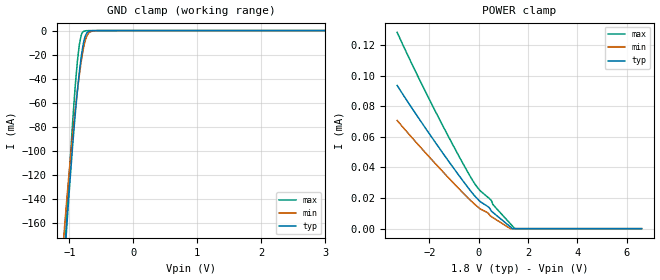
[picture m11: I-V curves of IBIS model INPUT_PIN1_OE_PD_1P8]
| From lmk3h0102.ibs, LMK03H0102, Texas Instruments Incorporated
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[Model]   INPUT_PIN1_OE_PD_1P8
Model_type   Input
Vinl = 0.65
Vinh = 1.15
|   typ   min   max
C_comp   0.7pF   0.5pF   0.9pF
[Voltage Range]   1.8   1.71   1.89
[Temperature Range]   45   125   -40
[Power Clamp Reference]   1.8   1.71   1.89
[GND Clamp Reference]   0   0   0
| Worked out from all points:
|   GND clamp passes 1 mA (typ) near -0.71 V on its own axis
[GND Clamp]
|   Voltage   I(typ)   I(min)   I(max)
-3.3V     -2.163A    -1.946A    -2.393A
-1.142V   -244.3mA   -209.2mA   -247.1mA
-1.073V   -188.3mA   -161.6mA   -183.1mA
-1.043V   -165mA     -142.2mA   -156.3mA
-943.8mV  -92.69mA   -84.35mA   -72.63mA
-874.5mV  -50.33mA   -50.21mA   -25.69mA
-844.8mV  -35.17mA   -37.37mA   -12.01mA
-815.1mV  -22.23mA   -25.95mA   -4.039mA
-765.6mV  -7.235mA   -11.31mA   -401.3uA
-696.3mV  -683.6uA   -2.04mA    -32.8uA
-577.5mV  -20.36uA   -85.13uA   -17.77uA
6.6V      0A         0A         0A
[POWER Clamp]
|   Voltage   I(typ)   I(min)   I(max)
-3.3V     93.64uA    70.75uA    128.4uA
-2.458V   72.96uA    55.1uA     99.55uA
-1.785V   57.13uA    43.09uA    77.77uA
-815.1mV  35.17uA    26.39uA    47.91uA
-260.7mV  23.38uA    17.42uA    32.01uA
36.3mV    18.09uA    13.27uA    25.25uA
412.5mV   13.97uA    9.645uA    20.01uA
491.7mV   12.08uA    8.166uA    18.83uA
600.6mV   10.32uA    6.999uA    15.4uA
1.284V    1.22uA     13.22nA    3.252uA
1.462V    0A         0A         96.92nA
6.6V      0A         0A         0A
